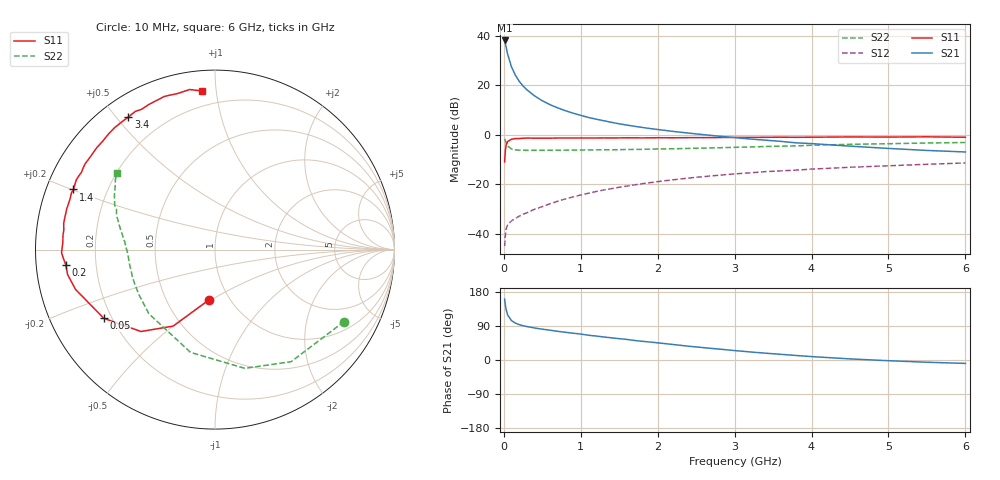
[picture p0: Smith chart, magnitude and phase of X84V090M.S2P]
! SIEMENS Small Signal Semiconductors
! BFP136W
! Si NPN RF Bipolar Junction Transistor in SOT343
! VCE = 4 V  IC = 90 mA
! Common Emitter S-Parameters:  September  1994
# GHz  S  MA  R  50
!  f  S11  S21  S12  S22
! GHz  MAG  ANG  MAG  ANG  MAG  ANG  MAG  ANG
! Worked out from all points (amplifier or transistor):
!   40 points, 10 MHz to 6 GHz, reference 50 ohm
!   highest |S21| = 38.0 dB at 10 MHz (marker M1)
!   |S21| within 3 dB of that: start of sweep to 32.03 MHz
!   unconditionally stable (mu >= 1): 533.9 MHz to 2.902 GHz
!   at 200 MHz: K = 0.67, MSG = 27.2 dB, |S12| = -32.9 dB
!   at 1.5 GHz: K = 1.10, MAG = 10.9 dB, |S12| = -21.2 dB
!   at 6 GHz: K = 0.97, MSG = 2.2 dB, |S12| = -11.4 dB
!   S11 on the Smith chart (normalised r, x): 10 MHz: 0.80, -0.49; 50 MHz: 0.17, -0.28; 200 MHz: 0.09, -0.05; 1.4 GHz: 0.08, +0.20; 3.4 GHz: 0.08, +0.54; 6 GHz: 0.11, +0.92
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0.01  0.2819 -96.9  79.84 160.7  0.0056 71.0  0.8238 -29.1
0.02  0.4852 -118.6  69.04 144.5  0.0095 57.3  0.755 -55.8
0.03  0.615 -132.1  58.45 132.9  0.0125 50.5  0.6821 -75.9
0.05  0.7285 -148.3  41.95 118.6  0.0153 40.1  0.5886 -103.4
0.1  0.8082 -164.1  23.28 103.9  0.0182 35.2  0.5132 -135.9
0.15  0.833 -170.4  15.85 97.3  0.0203 37.7  0.4924 -149.6
0.2  0.8357 -174.2  11.92 93.3  0.0226 40.2  0.4863 -157.0
0.25  0.8469 -176.9  9.614 90.5  0.0247 43.4  0.4845 -161.8
0.3  0.8551 -178.8  8.048 88.3  0.0265 46.2  0.4823 -165.0
0.4  0.8488 177.3  6.054 84.5  0.0312 50.4  0.4828 -169.3
0.5  0.8507 174.6  4.835 81.3  0.0353 53.5  0.4832 -172.1
0.6  0.8496 172.6  4.029 78.7  0.0402 55.7  0.4841 -174.0
0.7  0.8558 170.1  3.473 75.6  0.0453 57.8  0.4852 -175.4
0.9  0.8555 166.6  2.717 70.7  0.0553 59.3  0.4878 -178.0
1.1  0.8553 162.1  2.224 65.3  0.0656 60.2  0.4913 -179.7
1.4  0.8573 157.0  1.774 58.5  0.0814 60.0  0.4954 177.9
2.2  0.8659 143.1  1.163 40.9  0.1226 54.9  0.5185 171.9
3.2  0.881 126.1  0.817 21.3  0.1696 45.8  0.564 163.2
3.4  0.8826 123.1  0.774 18.0  0.1791 43.8  0.5772 161.4
4.5  0.8989 108.2  0.586 2.9  0.2195 33.6  0.6372 151.6
5.5  0.9029 99.0  0.48 -5.9  0.2521 25.8  0.6782 144.9
6  0.8865 94.6  0.447 -9.0  0.2683 21.5  0.694 141.9
